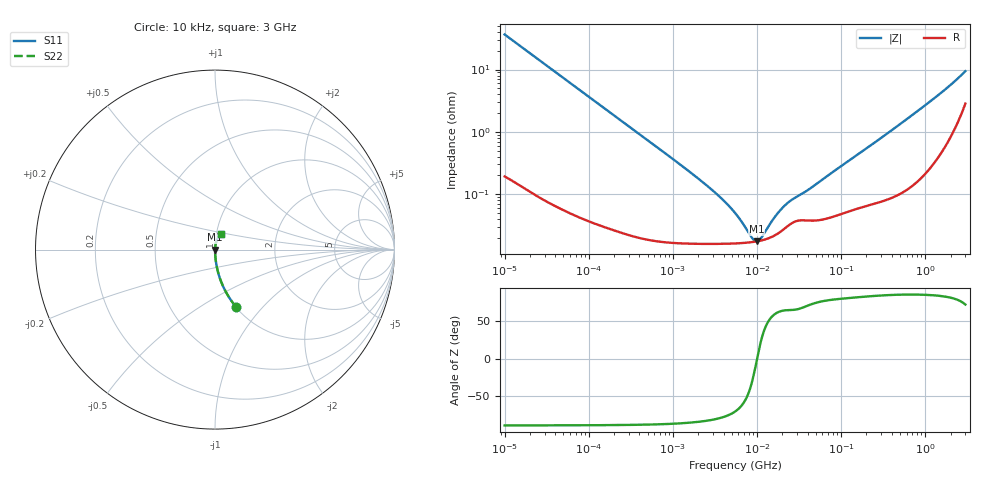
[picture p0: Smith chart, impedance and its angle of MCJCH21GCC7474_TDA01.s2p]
! MCJCH21GCC7474_TDA01  S-PARAMETER MODEL  ( Standard Model )
! Model Generated by TAIYO YUDEN Corporation (http://www.ty-top.com)
! Version 1.0
! TAIYO YUDEN Control No. 220601
! Copyright(c) 2016 TAIYO YUDEN CO.,LTD. All Rights Reserved.
! Product Description (link to TY-COMPAS)
! https://ds.yuden.co.jp/TYCOMPAS/or/detail?pn=MCJCH21GCC7474KTDA01&u=M
! Products Name : Multilayer Ceramic Capacitors
! Characteristics :
!  Capacitance : 0.47 [uF] , Rated Voltage : 100 [V] , TCC : X7S
!  Case Size : 2.0 x 1.25 / 0.079 x 0.049 [mm/inch] , Thickness : 1.25 / 0.049 [mm/inch]
!  (Conditions: Temperature = 25 [degC] , DC Bias Voltage = 0 [V])
! External Node Assignments :
!  1  o---| |---o  2
! GND o---------o GND
! Frequency Range : 10kHz  -  3GHz  [ 401 STEP ]
# MHZ S RI R 50
! Freq[MHz].  S11 Real  S11 Imag  S21 Real  S21 Imag  S12 Real  S12 Imag  S22 Real  S22 Imag
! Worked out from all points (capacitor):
!   401 points, 10 kHz to 3 GHz, reference 50 ohm
!   read as one part in series: C = 436 nF near 10.65 kHz
!   lowest |Z| = 17.6 mohm at 9.971 MHz (marker M1)
!   series resonance near 10.03 MHz, so ESL is about 580 pH
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0.01  0.1187 -0.3208  0.8813 0.3208  0.8813 0.3208  0.1187 -0.3208
0.015549  0.0535 -0.2221  0.9465 0.2221  0.9465 0.2221  0.0535 -0.2221
0.026575  0.0194 -0.1349  0.9806 0.1349  0.9806 0.1349  0.0194 -0.1349
0.045421  0.00705 -0.0801  0.9929 0.0801  0.9929 0.0801  0.00705 -0.0801
0.082683  0.00238 -0.0443  0.9976 0.0443  0.9976 0.0443  0.00238 -0.0443
0.683653  0.000203 -0.00539  0.9998 0.00539  0.9998 0.00539  0.000203 -0.00539
2.737278  0.000161 -0.00125  0.9998 0.00125  0.9998 0.00125  0.000161 -0.00125
3.996065  0.000161 -0.000781  0.9998 0.000781  0.9998 0.000781  0.000161 -0.000781
5.477226  0.000163 -0.000476  0.9998 0.000476  0.9998 0.000476  0.000163 -0.000476
6.617858  0.000165 -0.000317  0.9998 0.000317  0.9998 0.000317  0.000165 -0.000317
8.789267  0.000171 -9.86e-05  0.9998 9.86e-05  0.9998 9.86e-05  0.000171 -9.86e-05
9.361346  0.000173 -5.16e-05  0.9998 5.16e-05  0.9998 5.16e-05  0.000173 -5.16e-05
9.97066  0.000175 -4.71e-06  0.9998 4.71e-06  0.9998 4.71e-06  0.000175 -4.71e-06
10.61963  0.000178 4.22e-05  0.9998 -4.22e-05  0.9998 -4.22e-05  0.000178 4.22e-05
11.31085  0.000182 8.93e-05  0.9998 -8.93e-05  0.9998 -8.93e-05  0.000182 8.93e-05
15.99985  0.000216 0.000358  0.9998 -0.000358  0.9998 -0.000358  0.000216 0.000358
21.24962  0.000281 0.00059  0.9997 -0.00059  0.9997 -0.00059  0.000281 0.00059
25.67485  0.00034 0.000732  0.9997 -0.000732  0.9997 -0.000732  0.00034 0.000732
45.28751  0.000378 0.00125  0.9996 -0.00125  0.9996 -0.00125  0.000378 0.00125
374.4521  0.000942 0.00991  0.9991 -0.00991  0.9991 -0.00991  0.000942 0.00991
1280.606  0.00435 0.0342  0.9956 -0.0342  0.9956 -0.0342  0.00435 0.0342
3000  0.035 0.0843  0.965 -0.0843  0.965 -0.0843  0.035 0.0843
